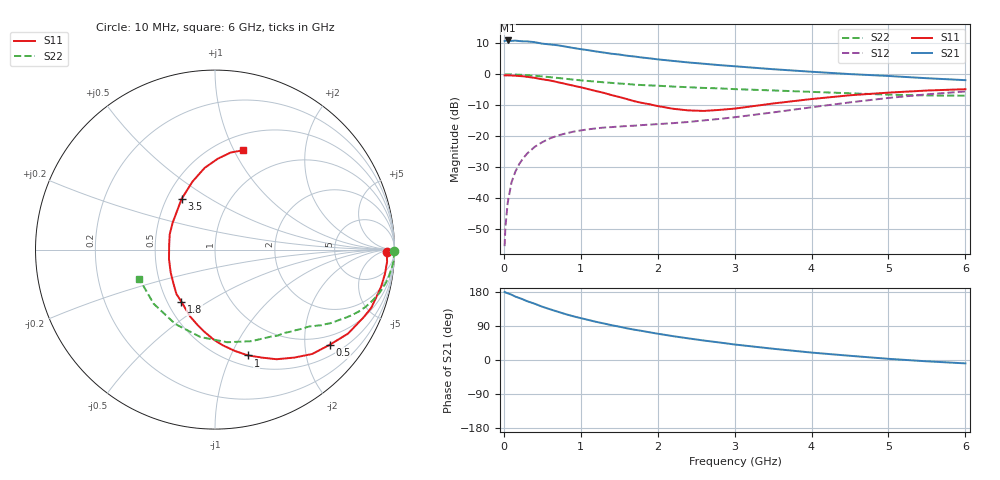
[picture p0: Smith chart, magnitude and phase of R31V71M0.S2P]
! SIEMENS Small Signal Semiconductors
! BFR181
! Si NPN RF Bipolar Junction Transistor in SOT23
! VCE = 1.75 V  IC = 1 mA
! Common Emitter S-Parameters:  May  1996
# GHz  S  MA  R  50
!  f  S11  S21  S12  S22
! GHz  MAG  ANG  MAG  ANG  MAG  ANG  MAG  ANG
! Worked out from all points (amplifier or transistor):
!   36 points, 10 MHz to 6 GHz, reference 50 ohm
!   highest |S21| = 10.9 dB at 50 MHz (marker M1)
!   |S21| within 3 dB of that: start of sweep to 1.057 GHz
!   unconditionally stable (mu >= 1): 1.982 GHz to 3.704 GHz
!   at 250 MHz: K = 0.15, MSG = 18.9 dB, |S12| = -27.1 dB
!   at 1.4 GHz: K = 0.78, MSG = 11.8 dB, |S12| = -17.0 dB
!   at 6 GHz: K = 0.89, MSG = 1.8 dB, |S12| = -5.5 dB
!   S11 on the Smith chart (normalised r, x): 10 MHz: 44, -15; 500 MHz: 0.75, -2.58; 1 GHz: 0.61, -1.16; 1.8 GHz: 0.59, -0.39; 3.5 GHz: 0.60, +0.38; 6 GHz: 0.66, +1.09
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0.01  0.9599 -0.8  3.428 179.6  0.0017 93.7  0.9989 -0.4
0.02  0.9576 -1.6  3.463 178.3  0.0034 89.7  0.9934 -0.8
0.05  0.9612 -4.0  3.507 176.1  0.0085 88.9  0.9974 -2.0
0.1  0.9563 -8.3  3.447 172.4  0.0182 84.4  0.996 -3.9
0.15  0.9484 -12.6  3.489 167.3  0.027 81.1  0.99 -5.9
0.2  0.9376 -16.2  3.431 163.7  0.0358 79.5  0.9831 -7.7
0.3  0.9103 -24.4  3.392 155.4  0.0524 74.2  0.9681 -11.3
0.4  0.8765 -32.3  3.293 148.5  0.0676 69.6  0.9483 -14.7
0.5  0.8303 -39.7  3.114 140.6  0.0806 64.9  0.9229 -17.9
0.7  0.7464 -53.7  2.935 127.5  0.103 57.8  0.8733 -23.2
0.8  0.7004 -60.7  2.796 121.2  0.1111 54.6  0.8466 -25.5
1  0.6175 -72.7  2.539 110.5  0.1245 49.7  0.7981 -29.3
1.1  0.5754 -78.9  2.442 105.6  0.1298 47.8  0.7793 -31.0
1.4  0.462 -97.3  2.142 91.9  0.1409 43.8  0.7262 -35.5
1.6  0.3985 -110.2  1.991 83.6  0.1465 42.9  0.6973 -37.7
1.8  0.3454 -122.8  1.859 76.6  0.1519 43.1  0.6703 -40.1
2.2  0.2781 -152.7  1.642 62.9  0.1632 44.5  0.6339 -45.2
3  0.2797 147.5  1.347 40.9  0.2032 49.4  0.5763 -57.3
3.5  0.3382 123.4  1.207 29.7  0.2431 50.5  0.5491 -68.3
4.5  0.4591 97.2  1.007 11.1  0.3527 45.9  0.494 -99.4
5.5  0.5474 80.9  0.864 -3.5  0.475 33.3  0.4559 -138.6
6  0.5753 74.2  0.804 -8.9  0.5287 25.5  0.4522 -159.1
